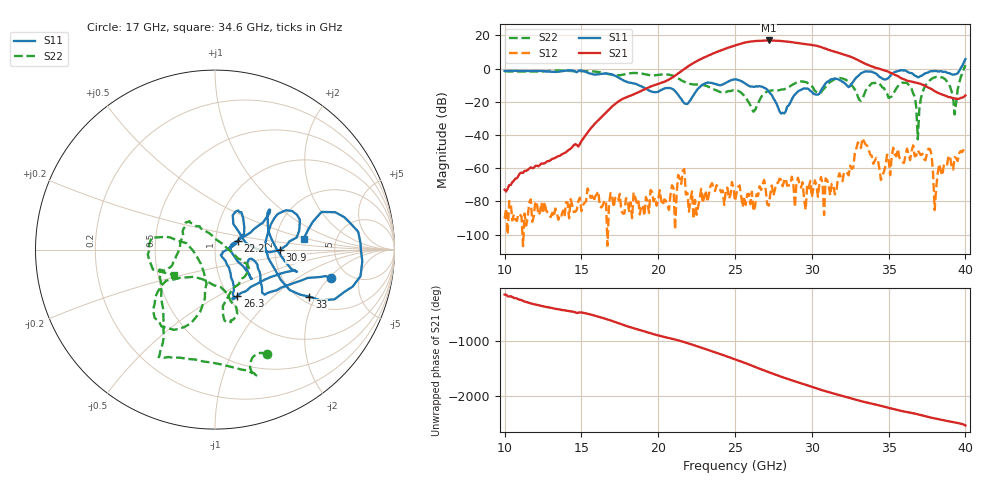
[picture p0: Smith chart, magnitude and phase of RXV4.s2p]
!Keysight Technologies,M9808A,MY58100618,A.14.70.03
!Date: Monday, February 27, 2023 13:25:51
!Correction: S11(Cdelta 2-Port  )
!S21(Cdelta 2-Port  )
!S12(Cdelta 2-Port  )
!S22(Cdelta 2-Port  )
!S2P File: Measurements: S11, S21, S12, S22:
# Hz S  RI  R 50
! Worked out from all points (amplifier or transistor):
!   301 points, 10 GHz to 40 GHz, reference 50 ohm
!   highest |S21| = 16.9 dB at 27.2 GHz (marker M1)
!   |S21| within 3 dB of that: 25.01 GHz to 30.18 GHz (5.175 GHz wide, 18.8 % of centre)
!   unconditionally stable (mu >= 1): start of sweep to 39.64 GHz
!   at 15 GHz: K = 108644.11, MAG = -32.3 dB, |S12| = -85.8 dB
!   at 25 GHz: K = 735.24, MAG = 15.2 dB, |S12| = -79.9 dB
!   at 40 GHz: K = 1392.50, MSG = 16.1 dB, |S12| = -48.3 dB
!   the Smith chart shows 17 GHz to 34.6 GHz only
!   S11 on the Smith chart (normalised r, x): 17 GHz: 3.72, -2.09; 22.2 GHz: 1.28, +0.13; 26.3 GHz: 1.10, -0.62; 30.9 GHz: 2.13, -0.01; 33 GHz: 2.23, -1.78; 34.6 GHz: 2.90, +0.45
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1e10  0.1533 0.837  -0.000189 -0.000123  -2.7e-05 -1.36e-05  0.7088 0.4319
1.5e10  0.6878 0.5398  -0.00262 -0.00596  2.58e-05 -4.42e-05  0.633 -0.5405
1.7e10  0.6458 -0.1568  -0.00377 0.0722  -0.0001 0.000101  0.2923 -0.5789
2e10  0.1775 -0.0933  -0.3434 -0.0538  -9.09e-05 7.23e-05  -0.2308 -0.6018
2.22e10  0.1255 0.0496  1.284 0.54  0.000157 0.000124  -0.3059 -0.1449
2.37e10  0.2911 0.1885  -1.368 -2.687  -2.66e-05 0.000204  -0.2216 -0.055
2.44e10  0.369 -0.0369  -3.99 0.3654  3.42e-05 0.000207  -0.1769 0.081
2.5e10  0.4568 -0.1226  -2.107 4.49  -6.43e-05 -7.83e-05  -0.1575 0.153
2.56e10  0.3428 -0.142  3.613 4.811  8.83e-05 0.000106  -0.0852 0.1296
2.63e10  0.1241 -0.2575  6.124 -2.819  -4.89e-05 4.84e-05  0.048 0.0287
2.68e10  0.1045 -0.2624  1.382 -6.763  -0.000338 -1.67e-05  0.1488 -0.0572
2.72e10  0.0991 -0.1775  -3.509 -6.09  5.7e-05 4.82e-05  0.1865 -0.097
2.78e10  0.0472 -0.0496  -6.88 0.2574  0.000358 6.73e-05  0.1511 -0.161
2.86e10  0.093 0.014  -1.214 6.204  0.00016 -0.000267  0.0568 -0.2908
2.93e10  0.1583 0.1658  4.53 3.509  0.000245 -9.2e-05  0.0901 -0.4033
3e10  0.1002 0.1748  4.652 -2.189  -0.000101 -8.89e-05  0.0862 -0.2855
3.09e10  0.3606 -0.00195  -1.12 -3.828  0.000489 9.06e-05  -0.2264 -0.166
3.18e10  0.3953 0.2192  -2.919 -0.1468  -0.000611 -0.000359  -0.2985 -0.4282
3.3e10  0.5253 -0.2616  0.078 1.81  0.00225 -0.00555  -0.0617 -0.1283
3.46e10  0.4936 0.0589  0.8686 -0.303  -0.000323 0.00047  -0.2293 -0.1418
3.5e10  0.478 -0.2199  0.5353 -0.5839  0.00103 -0.00166  0.0102 -0.131
4e10  1.142 -1.546  0.1543 -0.0247  -0.0006 -0.00381  0.5743 -1.138
